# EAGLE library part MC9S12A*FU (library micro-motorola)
MC9S12A256 microcontroller unit (MCU) 16-bit HCS12 Core; Upward compatible with M68HC11 instruction set Source: 9S12A128DGV1.pdf; 9S12A256DGV1.pdf
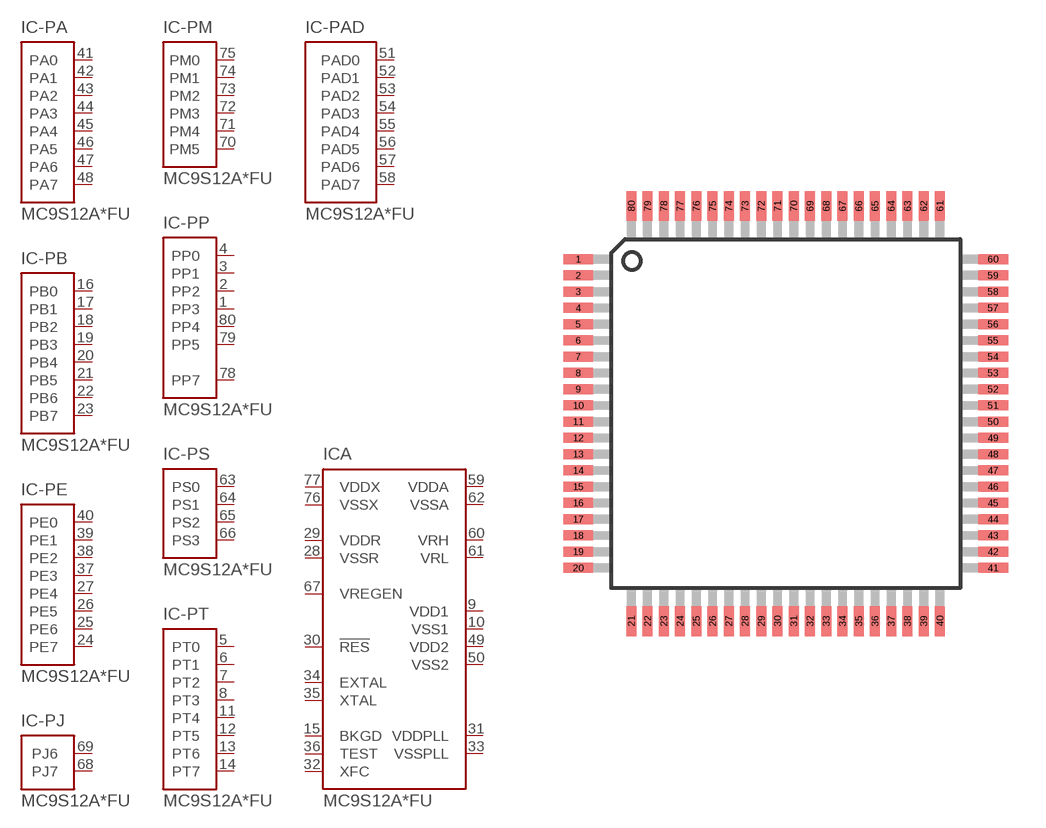
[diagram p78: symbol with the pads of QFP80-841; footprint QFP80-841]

Designator prefix IC; gates -PT=MC9S12-PT -PB=MC9S12-PB -PE=MC9S12-PE A=MC9S12A256 -PM=MC9S12-PM-80 -PS=MC9S12-PS-80 -PAD=MC9S12-PADAN0 -PP=MC9S12-PP-80 -PA=MC9S12-PA -PJ=MC9S12-PJ-80

## MC9S12A128BCFU (MF: MOTOROLA; MPN: MC9S12A128CFU; OC_FARNELL: 8686688; OC_NEWARK: 86H4600), MC9S12A256CFU (MPN: MC9S12A256CFU; OC_FARNELL: 1165784; OC_NEWARK: 62K5176)  [QFP80-841]
1  -PP:PP3
2  -PP:PP2
3  -PP:PP1
4  -PP:PP0
5  -PT:PT0
6  -PT:PT1
7  -PT:PT2
8  -PT:PT3
9  A:VDD1  out
10  A:VSS1  out
11  -PT:PT4
12  -PT:PT5
13  -PT:PT6
14  -PT:PT7
15  A:BKGD  oc
16  -PB:PB0
17  -PB:PB1
18  -PB:PB2
19  -PB:PB3
20  -PB:PB4
21  -PB:PB5
22  -PB:PB6
23  -PB:PB7
24  -PE:PE7
25  -PE:PE6
26  -PE:PE5
27  -PE:PE4
28  A:VSSR  pwr
29  A:VDDR  pwr
30  A:!RES
31  A:VDDPLL  out
32  A:XFC
33  A:VSSPLL  out
34  A:EXTAL  in
35  A:XTAL  out
36  A:TEST  in
37  -PE:PE3
38  -PE:PE2
39  -PE:PE1  in
40  -PE:PE0  in
41  -PA:PA0
42  -PA:PA1
43  -PA:PA2
44  -PA:PA3
45  -PA:PA4
46  -PA:PA5
47  -PA:PA6
48  -PA:PA7
49  A:VDD2  out
50  A:VSS2  out
51  -PAD:PAD0
52  -PAD:PAD1
53  -PAD:PAD2
54  -PAD:PAD3
55  -PAD:PAD4
56  -PAD:PAD5
57  -PAD:PAD6
58  -PAD:PAD7
59  A:VDDA  pwr
60  A:VRH  in
61  A:VRL  in
62  A:VSSA  pwr
63  -PS:PS0
64  -PS:PS1
65  -PS:PS2
66  -PS:PS3
67  A:VREGEN  in
68  -PJ:PJ7
69  -PJ:PJ6
70  -PM:PM5
71  -PM:PM4
72  -PM:PM3
73  -PM:PM2
74  -PM:PM1
75  -PM:PM0
76  A:VSSX  pwr
77  A:VDDX  pwr
78  -PP:PP7
79  -PP:PP5
80  -PP:PP4

## Footprint QFP80-841 (pad centres in mm)
80-Pin QFP (Case no. 841B) 9S12A256DGV1.pdf
smd 1.2 x 0.4: 1 -8.3,6.175; 2 -8.3,5.525; 3 -8.3,4.875; 4 -8.3,4.225; 5 -8.3,3.575; 6 -8.3,2.925; 7 -8.3,2.275; 8 -8.3,1.625; 9 -8.3,0.975; 10 -8.3,0.325; 11 -8.3,-0.325; 12 -8.3,-0.975; 13 -8.3,-1.625; 14 -8.3,-2.275; 15 -8.3,-2.925; 16 -8.3,-3.575; 17 -8.3,-4.225; 18 -8.3,-4.875; 19 -8.3,-5.525; 20 -8.3,-6.175; 41 8.3,-6.175; 42 8.3,-5.525; 43 8.3,-4.875; 44 8.3,-4.225; 45 8.3,-3.575; 46 8.3,-2.925; 47 8.3,-2.275; 48 8.3,-1.625; 49 8.3,-0.975; 50 8.3,-0.325; 51 8.3,0.325; 52 8.3,0.975; 53 8.3,1.625; 54 8.3,2.275; 55 8.3,2.925; 56 8.3,3.575; 57 8.3,4.225; 58 8.3,4.875; 59 8.3,5.525; 60 8.3,6.175
smd 0.4 x 1.2: 21 -6.175,-8.3; 22 -5.525,-8.3; 23 -4.875,-8.3; 24 -4.225,-8.3; 25 -3.575,-8.3; 26 -2.925,-8.3; 27 -2.275,-8.3; 28 -1.625,-8.3; 29 -0.975,-8.3; 30 -0.325,-8.3; 31 0.325,-8.3; 32 0.975,-8.3; 33 1.625,-8.3; 34 2.275,-8.3; 35 2.925,-8.3; 36 3.575,-8.3; 37 4.225,-8.3; 38 4.875,-8.3; 39 5.525,-8.3; 40 6.175,-8.3; 61 6.175,8.3; 62 5.525,8.3; 63 4.875,8.3; 64 4.225,8.3; 65 3.575,8.3; 66 2.925,8.3; 67 2.275,8.3; 68 1.625,8.3; 69 0.975,8.3; 70 0.325,8.3; 71 -0.325,8.3; 72 -0.975,8.3; 73 -1.625,8.3; 74 -2.275,8.3; 75 -2.925,8.3; 76 -3.575,8.3; 77 -4.225,8.3; 78 -4.875,8.3; 79 -5.525,8.3; 80 -6.175,8.3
